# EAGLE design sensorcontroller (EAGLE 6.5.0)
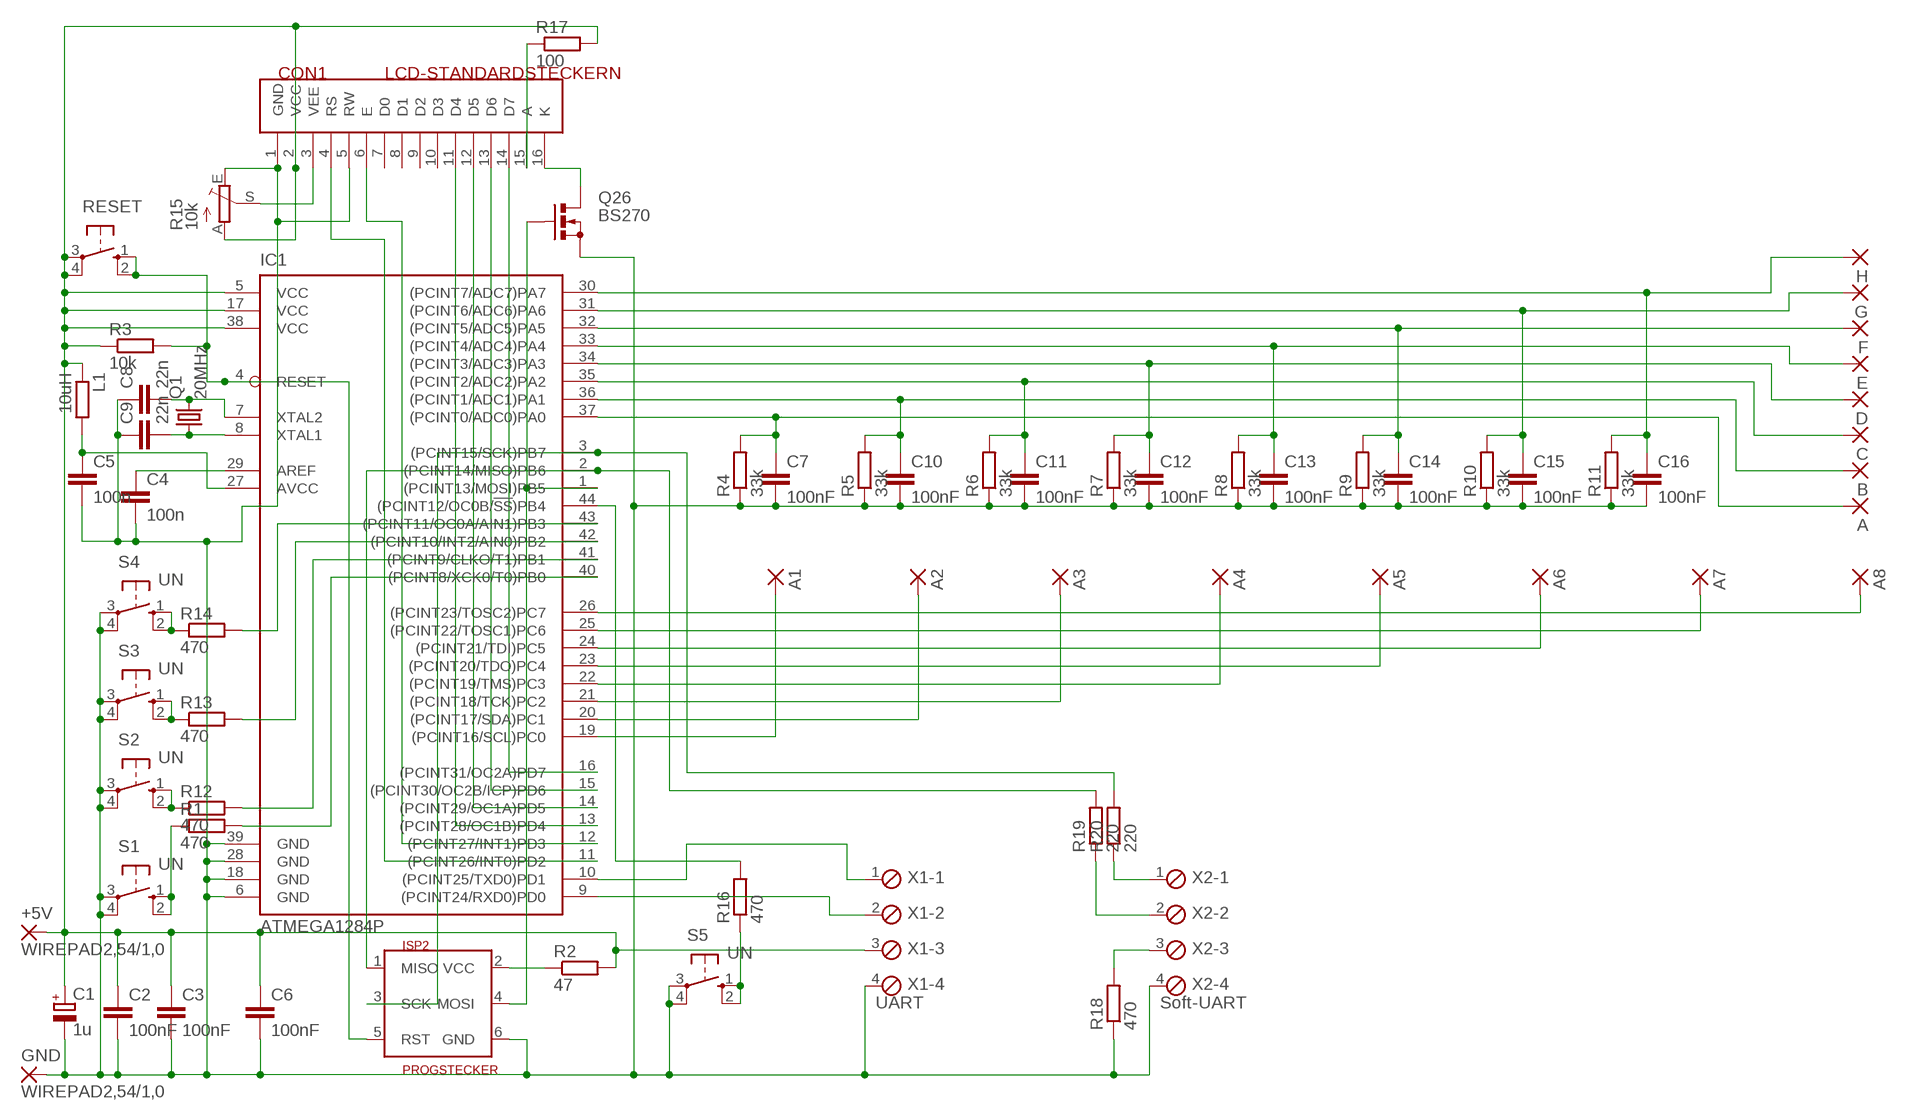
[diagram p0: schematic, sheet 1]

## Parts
+5V  WIREPAD2,54/1,0  [2,54/1,0]
A  WIREPAD2,15/1,0  [2,15/1,0]
A1  WIREPAD2,15/1,0  [2,15/1,0]
A2  WIREPAD2,15/1,0  [2,15/1,0]
A3  WIREPAD2,15/1,0  [2,15/1,0]
A4  WIREPAD2,15/1,0  [2,15/1,0]
A5  WIREPAD2,15/1,0  [2,15/1,0]
A6  WIREPAD2,15/1,0  [2,15/1,0]
A7  WIREPAD2,15/1,0  [2,15/1,0]
A8  WIREPAD2,15/1,0  [2,15/1,0]
B  WIREPAD2,15/1,0  [2,15/1,0]
C  WIREPAD2,15/1,0  [2,15/1,0]
C1  1u  CPOL-EUE5-6  [E5-6]
C2  100nF  C-EU025-025X050  [C025-025X050]
C3  100nF  C-EU025-025X050  [C025-025X050]
C4  100n  C-EUC1206  [C1206]
C5  100n  C-EUC1206  [C1206]
C6  100nF  C-EU025-025X050  [C025-025X050]
C7  100nF  C-EUC1206  [C1206]
C8  22n  C-EUC1206  [C1206]
C9  22n  C-EUC1206  [C1206]
C10  100nF  C-EUC1206  [C1206]
C11  100nF  C-EUC1206  [C1206]
C12  100nF  C-EUC1206  [C1206]
C13  100nF  C-EUC1206  [C1206]
C14  100nF  C-EUC1206  [C1206]
C15  100nF  C-EUC1206  [C1206]
C16  100nF  C-EUC1206  [C1206]
CON1  LCD-STANDARDSTECKERN  [STECKER16]
D  WIREPAD2,15/1,0  [2,15/1,0]
E  WIREPAD2,15/1,0  [2,15/1,0]
F  WIREPAD2,15/1,0  [2,15/1,0]
G  WIREPAD2,15/1,0  [2,15/1,0]
GND  WIREPAD2,54/1,0  [2,54/1,0]
H  WIREPAD2,15/1,0  [2,15/1,0]
IC1  ATMEGA1284P  ATMEGA644A  [TQFP44]
ISP2  PROGSTECKER  ISP6N  [ISP6]
L1  10uH  R-EU_0204/7  [0204/7]
Q1  20MHz  CRYSTALHC49S  [HC49/S]
Q26  BS270  BS170  [SOT54E]
R1  470  R-EU_M1406  [M1406]
R2  47  R-EU_M1406  [M1406]
R3  10k  R-EU_M1406  [M1406]
R4  33k  R-EU_M1406  [M1406]
R5  33k  R-EU_M1406  [M1406]
R6  33k  R-EU_M1406  [M1406]
R7  33k  R-EU_M1406  [M1406]
R8  33k  R-EU_M1406  [M1406]
R9  33k  R-EU_M1406  [M1406]
R10  33k  R-EU_M1406  [M1406]
R11  33k  R-EU_M1406  [M1406]
R12  470  R-EU_M1406  [M1406]
R13  470  R-EU_M1406  [M1406]
R14  470  R-EU_M1406  [M1406]
R15  10k  TRIM_EU-CA6V  [CA6V]
R16  470  R-EU_M1406  [M1406]
R17  100  R-EU_0204/7  [0204/7]
R18  470  R-EU_M1406  [M1406]
R19  220  R-EU_M1406  [M1406]
R20  220  R-EU_M1406  [M1406]
RESET  10-XX  [B3F-10XX]
S1  UN  10-XX  [B3F-10XX]
S2  UN  10-XX  [B3F-10XX]
S3  UN  10-XX  [B3F-10XX]
S4  UN  10-XX  [B3F-10XX]
S5  UN  10-XX  [B3F-10XX]
X1  UART  MPT4  [4POL254]
X2  Soft-UART  MPT4  [4POL254]

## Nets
AVCC [dick]: C5.1 IC1.27(AVCC) L1.2
GND [dick]: C1.- C2.2 C3.2 C4.2 C5.2 C6.2 C7.2 C8.1 C9.1 C10.2 C11.2 C12.2 C13.2 C14.2 C15.2 C16.2 CON1.1(GND) CON1.5(RW) GND.1(P) IC1.6(GND) IC1.18(GND) IC1.28(GND) IC1.39(GND) ISP2.6(GND) Q26.S R4.1 R5.1 R6.1 R7.1 R8.1 R9.1 R10.1 R11.1 R15.E R18.1 S1.3(P) S1.4(P1) S2.3(P) S2.4(P1) S3.3(P) S3.4(P1) S4.3(P) S4.4(P1) S5.3(P) S5.4(P1) X1.4 X2.4
N$1: C8.2 IC1.7(XTAL2) Q1.2
N$2 [dick]: ISP2.2(VCC) R2.1
N$3: A.1(P) C7.1 IC1.37((PCINT0/ADC0)PA0) R4.2
N$4 [dick]: R1.1 S1.1(S) S1.2(S1)
N$5: C9.2 IC1.8(XTAL1) Q1.1
N$6: IC1.4(RESET) ISP2.5(RST) R3.2 RESET.1(S) RESET.2(S1)
N$7: C15.1 G.1(P) IC1.31((PCINT6/ADC6)PA6) R10.2
N$8: IC1.40((PCINT8/XCK0/T0)PB0) R1.2
N$9: B.1(P) C10.1 IC1.36((PCINT1/ADC1)PA1) R5.2
N$10 [dick]: C4.1 IC1.29(AREF)
N$11: A2.1(P) IC1.20((PCINT17/SDA)PC1)
N$12: IC1.1((PCINT13/MOSI)PB5) ISP2.4(MOSI) Q26.G
N$13 [dick]: R12.1 S2.1(S) S2.2(S1)
N$14: A3.1(P) IC1.21((PCINT18/TCK)PC2)
N$15: C14.1 F.1(P) IC1.32((PCINT5/ADC5)PA5) R9.2
N$16: C13.1 E.1(P) IC1.33((PCINT4/ADC4)PA4) R8.2
N$20: C12.1 D.1(P) IC1.34((PCINT3/ADC3)PA3) R7.2
N$21: A1.1(P) IC1.19((PCINT16/SCL)PC0)
N$25: C11.1 C.1(P) IC1.35((PCINT2/ADC2)PA2) R6.2
N$26: C16.1 H.1(P) IC1.30((PCINT7/ADC7)PA7) R11.2
N$27: A4.1(P) IC1.22((PCINT19/TMS)PC3)
N$31: A5.1(P) IC1.23((PCINT20/TDO)PC4)
N$35: A6.1(P) IC1.24((PCINT21/TDI)PC5)
N$39: A7.1(P) IC1.25((PCINT22/TOSC1)PC6)
N$43: A8.1(P) IC1.26((PCINT23/TOSC2)PC7)
N$52 [dick]: R13.1 S3.1(S) S3.2(S1)
N$53 [dick]: R14.1 S4.1(S) S4.2(S1)
N$54: IC1.41((PCINT9/CLKO/T1)PB1) R12.2
N$55: IC1.42((PCINT10/INT2/AIN0)PB2) R13.2
N$56: IC1.43((PCINT11/OC0A/AIN1)PB3) R14.2
N$57: CON1.3(VEE) R15.S
N$58: CON1.4(RS) IC1.11((PCINT26/INT0)PD2)
N$59: CON1.6(E) IC1.12((PCINT27/INT1)PD3)
N$60: CON1.11(D4) IC1.13((PCINT28/OC1B)PD4)
N$61: CON1.12(D5) IC1.14((PCINT29/OC1A)PD5)
N$62: CON1.13(D6) IC1.15((PCINT30/OC2B/ICP)PD6)
N$63: CON1.14(D7) IC1.16((PCINT31/OC2A)PD7)
N$64 [sehrdick]: CON1.16(K) Q26.D
N$65 [dick]: R16.1 S5.1(S) S5.2(S1)
N$66: IC1.44((PCINT12/OC0B/!SS!)PB4) R16.2
N$67 [sehrdick]: CON1.15(A) R17.1
N$68: IC1.9((PCINT24/RXD0)PD0) X1.2
N$69: IC1.10((PCINT25/TXD0)PD1) X1.1
N$70: R18.2 X2.3
N$71: R19.1 X2.2
N$72: R20.1 X2.1
RXD2: IC1.2((PCINT14/MISO)PB6) ISP2.1(MISO) R19.2
TXD2: IC1.3((PCINT15/SCK)PB7) ISP2.3(SCK) R20.2
VCC [dick]: +5V.1(P) C1.+ C2.1 C3.1 C6.1 CON1.2(VCC) IC1.5(VCC) IC1.17(VCC) IC1.38(VCC) L1.1 R2.2 R3.1 R15.A R17.2 RESET.3(P) RESET.4(P1) X1.3
Unconnected: CON1.7(D0) CON1.8(D1) CON1.9(D2) CON1.10(D3)

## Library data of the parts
+5V A A1-A8 B C D E F G GND H = wirepad:WIREPAD: Wire PAD connect wire on PCB
C1 = resistor:CPOL-EU: POLARIZED CAPACITOR, European symbol
C2-C16 = rcl:C-EU: CAPACITOR, European symbol
CON1 = 6_stecker:LCD-STANDARDSTECKER: Standard-Stecker fuer die meisten LCD-Module
IC1 = atmel:ATMEGA644: 8-bit Microcontroller with 64K Bytes In-System Programmable Flash Source: http://www.atmel.com/dyn/resources/prod_documents/doc2593.pdf; MPN: ATMEGA644PV-10AU; OC_FARNELL: 1455123; OC_NEWARK: 58M3748
ISP2 = stecker:ISP6: ISP-Stecker 6polig
L1 R1-R14 R16-R20 = rcl:R-EU_: RESISTOR, European symbol
Q1 = crystal:CRYSTAL: CRYSTAL
Q26 = transistor-small-signal:BS170: N-CHANNEL MOS FET
R15 = pot:TRIM_EU-: POTENTIOMETER
RESET S1-S5 = switch-omron:10-XX: OMRON SWITCH; MPN: B3F-1000; OC_FARNELL: 176432; OC_NEWARK: 36M3542
X1 X2 = con-phoenix-254:MPT4: PHOENIX CONNECTOR; OC_FARNELL: unknown; OC_NEWARK: unknown

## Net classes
1 dick: width 0.508 mm
2 sehrdick: width 1.016 mm

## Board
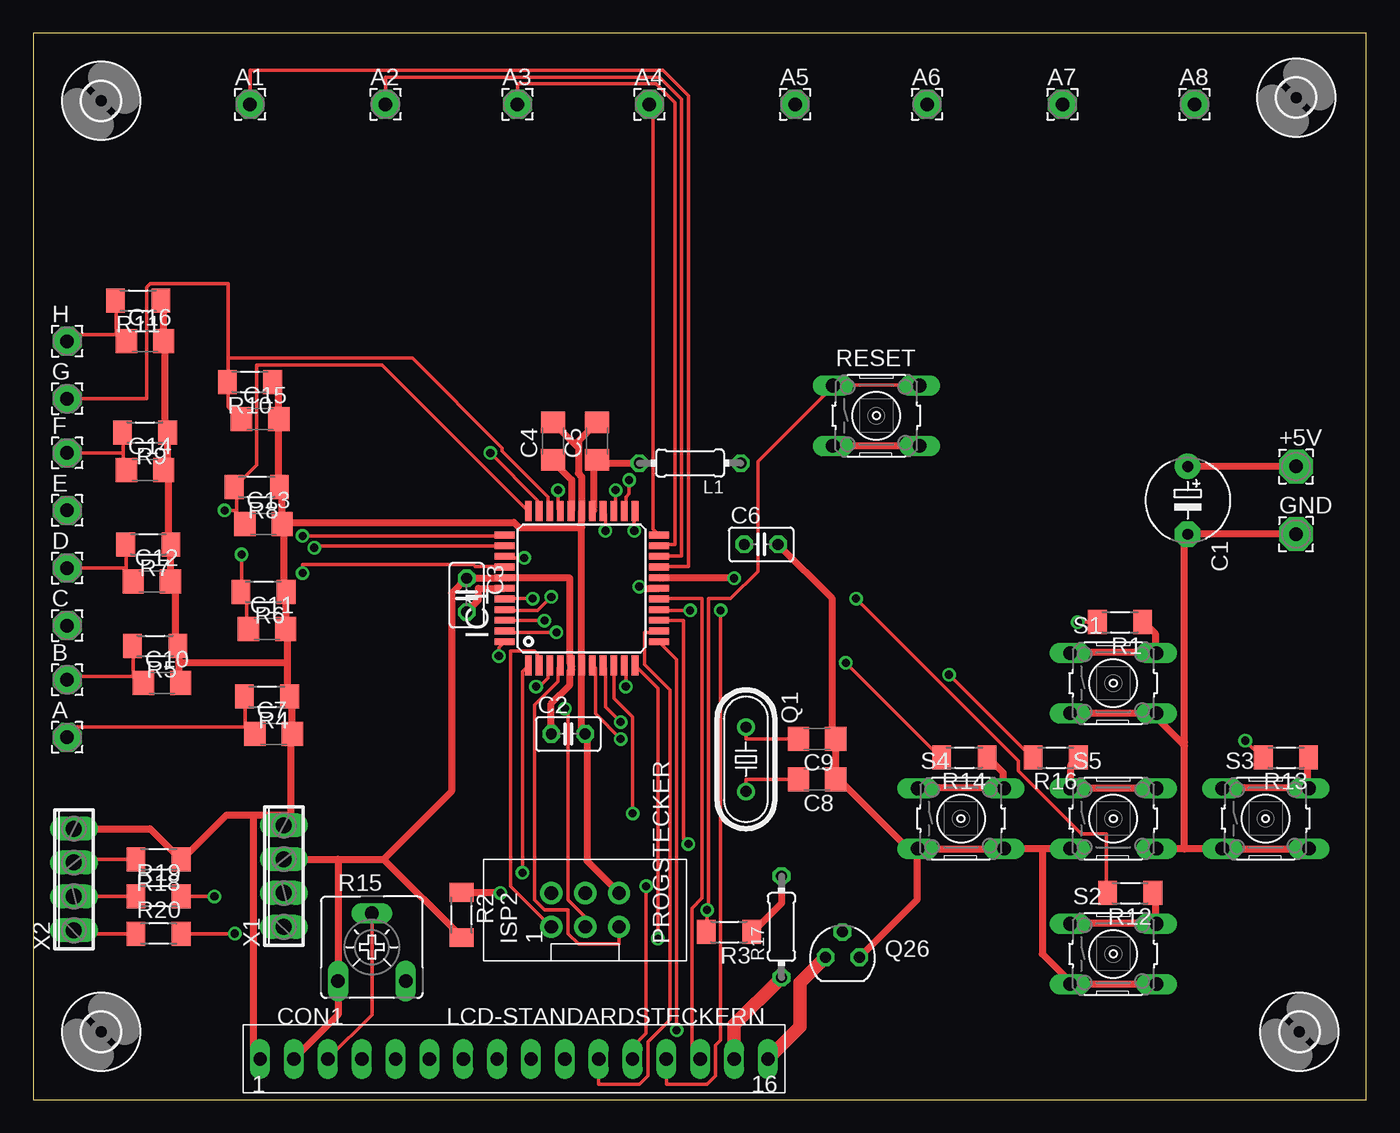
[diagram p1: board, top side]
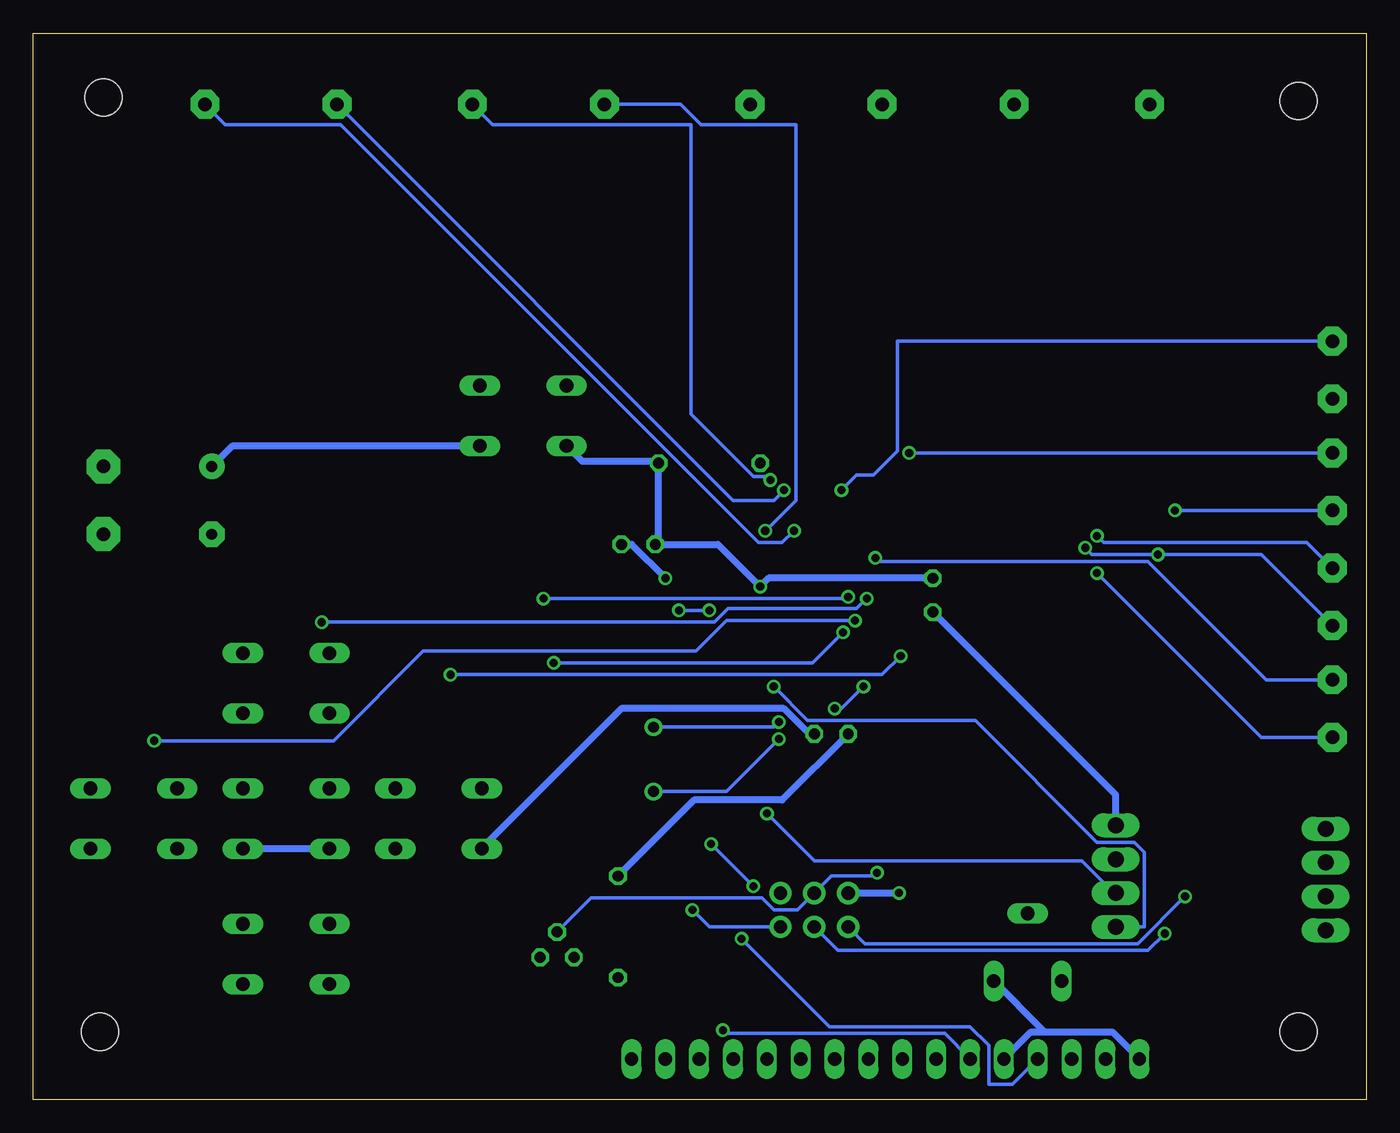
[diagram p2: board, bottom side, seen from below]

Size 100 x 80 mm. Coordinates in mm from the lower left corner, seen from the top.
Outline: 0,0 100,0 100,80 0,80 0,0
Copper layers (1*16): Top 0.035mm / dielectric 1.5mm / Bottom 0.035mm
Design rules "default": minimum track width 10mil, minimum drill 24mil, track to track 8mil, track to pad 8mil, pad to pad 8mil, via to via 8mil, smd to smd 8mil, copper to edge 40mil, drill to drill 8mil, minimum pad ring 10mil, minimum via ring 8mil, stop-mask expansion 4mil, vias tented up to drill 0mil, thermal gap 10mil

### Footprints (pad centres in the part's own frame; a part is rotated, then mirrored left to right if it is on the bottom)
2,54/1,0 = drill 1.016 pad 2.54 octagon: 1 0,0
2,15/1,0 = drill 1.016 pad 2.159 octagon: 1 0,0
E5-6 = drill 0.813 pad 1.905: + -2.54,0 | drill 0.813 pad 1.905 octagon: - 2.54,0
C025-025X050 = drill 0.813 octagon: 1 -1.27,0; 2 1.27,0
C1206 = smd 1.6 x 1.8: 1 -1.4,0; 2 1.4,0
STECKER16 = drill 1 long: 1 -17.78,0; 2 -15.24,0; 3 -12.7,0; 4 -10.16,0; 5 -7.62,0; 6 -5.08,0; 7 -2.54,0; 8 0,0; 9 2.54,0; 10 5.08,0; 11 7.62,0; 12 10.16,0; 13 12.7,0; 14 15.24,0; 15 17.78,0; 16 20.32,0
TQFP44 = smd 1.5 x 0.5: 1 -5.8,4; 2 -5.8,3.2; 3 -5.8,2.4; 4 -5.8,1.6; 5 -5.8,0.8; 6 -5.8,0; 7 -5.8,-0.8; 8 -5.8,-1.6; 9 -5.8,-2.4; 10 -5.8,-3.2; 11 -5.8,-4; 23 5.8,-4; 24 5.8,-3.2; 25 5.8,-2.4; 26 5.8,-1.6; 27 5.8,-0.8; 28 5.8,0; 29 5.8,0.8; 30 5.8,1.6; 31 5.8,2.4; 32 5.8,3.2; 33 5.8,4 | smd 0.5 x 1.5: 12 -4,-5.8; 13 -3.2,-5.8; 14 -2.4,-5.8; 15 -1.6,-5.8; 16 -0.8,-5.8; 17 0,-5.8; 18 0.8,-5.8; 19 1.6,-5.8; 20 2.4,-5.8; 21 3.2,-5.8; 22 4,-5.8; 34 4,5.8; 35 3.2,5.8; 36 2.4,5.8; 37 1.6,5.8; 38 0.8,5.8; 39 0,5.8; 40 -0.8,5.8; 41 -1.6,5.8; 42 -2.4,5.8; 43 -3.2,5.8; 44 -4,5.8
ISP6 = drill 1 pad 1.676: 1 -1.27,2.54; 2 1.27,2.54; 3 -1.27,0; 4 1.27,0; 5 -1.27,-2.54; 6 1.27,-2.54
0204/7 = drill 0.813 octagon: 1 -3.81,0; 2 3.81,0
HC49/S = drill 0.813: 1 -2.413,0; 2 2.413,0
SOT54E = drill 0.813 octagon: D -1.27,0; G 0,1.905; S 1.27,0
M1406 = smd 1.4 x 1.8: 1 -1.7,0; 2 1.7,0
CA6V = drill 1.016 long: A -2.54,-2.54; E 2.54,-2.54; S 0,2.54
B3F-10XX = drill 1.016 long: 1 -3.251,2.261; 2 3.251,2.261; 3 -3.251,-2.261; 4 3.251,-2.261
2,8 = hole 2.8: 0,0
4POL254 = drill 1.2 long: 1 -3.81,0; 2 -1.27,0; 3 1.27,0; 4 3.81,0

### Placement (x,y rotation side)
+5V  94.74,47.5 0 top
A  2.54,27.18 0 top
A1  16.26,74.68 0 top
A2  26.42,74.68 0 top
A3  36.32,74.68 0 top
A4  46.23,74.68 0 top
A5  57.15,74.68 0 top
A6  67.06,74.68 0 top
A7  77.22,74.68 0 top
A8  87.12,74.68 0 top
B  2.54,31.5 0 top
C  2.54,35.56 0 top
C1  86.61,44.96 270 top
C2  40.13,27.43 0 top
C3  32.51,37.85 270 top
C4  38.99,49.4 90 top
C5  42.29,49.4 90 top
C6  54.61,41.66 0 top
C7  18.03,27.43 0 top
C8  58.8,24 180 top
C9  58.8,27.05 180 top
C10  9.65,31.24 0 top
C11  17.53,35.31 0 top
C12  8.89,38.86 0 top
C13  17.27,43.18 0 top
C14  8.38,47.24 0 top
C15  17.02,51.05 0 top
C16  8.38,56.9 0 top
CON1  34.8,3.05 0 top
D  2.54,39.88 0 top
E  2.54,44.2 0 top
F  2.54,48.51 0 top
G  2.54,52.58 0 top
GND  94.74,42.42 0 top
H  2.54,56.9 0 top
IC1  41.15,38.35 90 top
ISP2  41.4,14.22 90 top
L1  49.28,47.75 180 top
Q1  53.47,25.53 270 top
Q26  60.71,10.67 0 top
R1  81.53,35.81 180 top
R2  32.13,13.84 270 top
R3  52.2,12.57 180 top
R4  17.53,30.23 180 top
R5  9.14,34.04 180 top
R6  17.27,38.1 180 top
R7  8.64,41.66 180 top
R8  16.76,45.97 180 top
R9  8.38,50.04 180 top
R10  16.26,53.85 180 top
R11  7.87,59.94 180 top
R12  82.3,15.49 180 top
R13  93.98,25.65 180 top
R14  69.85,25.65 180 top
R15  25.4,11.43 0 top
R16  76.71,25.65 180 top
R17  56.13,12.95 90 top
R18  9.4,18.03 180 top
R19  9.4,15.24 0 top
R20  9.4,12.45 0 top
RESET  63.25,51.31 0 top
S1  81.03,31.24 0 top
S2  81.03,10.92 0 top
S3  92.46,21.08 0 top
S4  69.6,21.08 0 top
S5  81.03,21.08 0 top
U$1  [2,8]  95,5.08 0 top
U$2  [2,8]  5.08,5.08 0 top
U$3  [2,8]  5.08,74.93 0 top
U$4  [2,8]  94.74,75.18 0 top
X1  18.8,16.76 90 top
X2  3.05,16.51 90 top

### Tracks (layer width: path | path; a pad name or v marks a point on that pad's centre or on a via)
AVCC
  Top 0.508: 42.04,44.2 IC1.27 42.04,44.45 42.04,47.62 42.29,47.88 C5.1 42.42,47.75 L1.2
GND  (via drill 0.61)
  Top 0.508: GND.1 C1.- 86.36,42.16 86.36,26.8 86.23,26.67 | S1.3 77.85,28.96 84.2,28.96 S1.4 84.2,28.7 86.23,26.67 | 86.36,18.8 89.15,18.8 S3.3 89.41,18.8 95.63,18.8 S3.4 | 86.36,18.8 84.33,18.8 S5.4 | 86.23,26.67 86.36,26.54 86.36,18.8 | 46.99,39.12 IC1.18 47.24,39.12 v52.58,39.12 | S2.4 84.2,8.64 77.85,8.64 S2.3 77.72,8.89 75.69,10.92 75.69,18.8 | 75.69,18.8 77.72,18.8 S5.3 | 75.69,18.8 72.9,18.8 S4.4 72.64,18.8 66.55,18.8 S4.3 | Q26.S 66.29,14.99 66.29,18.8 S4.3 | S4.3 66.17,18.29 60.45,24 C8.1 C9.1 60.07,27.18 59.94,27.3 59.94,37.59 C6.2 | 41.15,44.2 IC1.28 | IC1.28 41.15,46.74 40.89,46.99 40.89,49.02 | 40.89,49.02 40.89,49.4 C5.2 | C4.2 40.77,49.02 40.89,49.02 | 41.15,32.51 IC1.6 | IC1.6 41.15,27.69 C2.2 41.53,27.3 41.53,17.91 ISP2.6 | IC1.6 41.15,42.93 | 41.15,42.93 IC1.28 | R11.1 9.65,59.94 9.78,59.82 C16.2 9.91,56.77 9.91,50.16 R9.1 10.03,50.04 10.03,47.37 9.91,47.24 C14.2 10.03,47.12 10.16,46.99 10.16,41.78 R7.1 10.29,41.66 C12.2 10.41,38.73 10.67,38.48 10.67,34.16 R5.1 10.92,34.04 10.92,32.77 | 10.92,32.77 10.92,31.37 C10.2 | X2.4 8.76,20.32 11.05,18.03 R18.1 11.3,18.16 14.48,21.34 16.51,21.34 | 35.43,38.35 IC1.39 33.4,38.35 33.4,37.47 C3.2 | R10.1 18.03,53.85 18.41,53.47 C15.2 18.41,50.93 18.41,46.1 R8.1 18.54,45.97 18.67,45.85 C13.2 | C13.2 18.8,43.05 18.8,38.23 R6.1 18.92,38.1 C11.2 19.05,35.18 19.05,32.77 | 19.05,32.77 19.05,30.35 R4.1 19.3,30.23 19.43,30.1 C7.2 19.3,27.3 19.3,21.08 X1.4 19.18,21.34 16.51,21.34 | CON1.1 16.51,3.56 16.51,21.34 | 19.05,32.77 10.92,32.77 | 41.15,42.93 36.45,42.93 36.07,43.31 18.8,43.31 C13.2
  Bottom 0.508: v52.58,39.12 55.12,41.66 C6.2 | S5.4 84.2,18.8 77.85,18.8 S5.3 | CON1.1 19.05,5.08 24.26,5.08 | 24.26,5.08 25.15,5.08 CON1.5 | R15.E 24.26,5.21 24.26,5.08 | C3.2 18.8,22.86 X1.4 | C2.2 41.78,27.43 43.69,29.34 55.88,29.34 66.29,18.92 S4.3
N$1  (via drill 0.61)
  Top 0.254: v44.07,27.05 42.16,28.96 42.16,32.38 42.04,32.51 IC1.7 | C8.2 53.47,24 Q1.2
  Bottom 0.254: v44.07,27.05 48.01,23.11 Q1.2
N$2  (via drill 0.61)
  Top 0.508: v35.05,15.49 32.13,15.49 R2.1
  Bottom 0.508: ISP2.2 v35.05,15.49
N$3  (via drill 0.61)
  Top 0.254: R4.2 15.88,30.23 15.88,28.07 16.51,27.43 C7.1 15.88,27.94 2.54,27.94 A.1 | v20.19,39.5 20.19,40.13 33.02,40.13 33.15,40.01 35.31,40.01 IC1.37
  Bottom 0.254: v20.19,39.5 7.87,27.18 A.1
N$4
  Top 0.508: R1.1 83.31,35.81 84.2,34.92 84.2,33.53 S1.2 83.95,33.53 77.85,33.53 S1.1
N$5  (via drill 0.61)
  Top 0.254: v44.07,28.32 42.93,29.46 42.93,32.38 42.8,32.51 IC1.8 | C9.2 53.47,27.05 Q1.1
  Bottom 0.254: v44.07,28.32 44.45,27.94 Q1.1
N$6  (via drill 0.61)
  Top 0.254: RESET.2 66.42,53.59 60.07,53.59 RESET.1 59.94,53.47 54.36,47.88 54.36,39.62 52.32,37.59 50.67,37.59 50.67,14.35 v50.55,14.22 50.55,12.57 R3.2 | ISP2.5 43.94,11.68 40.89,11.68 40.13,12.45 40.13,14.22 38.35,14.22 37.59,14.99 37.59,29.59 39.37,31.37 39.37,32.38 39.5,32.51 IC1.4
  Bottom 0.254: v50.55,14.22 49.28,12.95 ISP2.5
N$7
  Top 0.254: 14.61,55.63 28.45,55.63 35.18,48.9 35.18,48.64 38.61,45.21 38.61,44.32 38.73,44.2 IC1.31 | 14.61,53.85 14.61,55.63 | 14.61,53.85 14.61,51.94 15.49,51.05 C15.1 | 14.61,53.85 R10.2 | G.1 8.51,52.58 8.51,60.96 8.76,61.21 14.61,61.21 14.61,55.63
N$8  (via drill 0.61)
  Top 0.254: v37.47,37.59 35.43,37.59 IC1.40 | R1.2 v78.36,35.81
  Bottom 0.254: v37.47,37.59 38.23,36.83 47.88,36.83 48.9,35.81 v78.36,35.81
N$9  (via drill 0.61)
  Top 0.254: R5.2 7.49,34.04 7.49,31.88 8.13,31.24 C10.1 7.49,31.75 2.54,31.75 B.1 | v36.83,40.64 35.43,40.64 IC1.36
  Bottom 0.254: v36.83,40.64 36.58,40.39 16.38,40.39 7.49,31.5 B.1
N$10
  Top 0.508: IC1.29 40.39,44.2 40.39,46.48 38.99,47.88 C4.1
N$11
  Top 0.254: A2.1 26.42,76.71 46.99,76.71 48.64,75.06 48.64,40.77 46.99,40.77 IC1.20
N$12  (via drill 0.61)
  Top 0.254: v36.7,17.02 36.7,32.13 37.08,32.51 IC1.1
  Bottom 0.254: v36.7,17.02 36.96,16.76 40.13,16.76 ISP2.4 42.67,14.22 44.45,14.22 45.34,15.11 58.17,15.11 Q26.G
N$13
  Top 0.508: R12.1 84.07,15.49 84.2,15.37 84.2,13.21 S2.2 83.95,13.21 77.85,13.21 S2.1
N$14
  Top 0.254: A3.1 36.32,76.2 46.74,76.2 48.13,74.8 48.13,41.66 46.99,41.66 IC1.21
N$15  (via drill 0.61)
  Top 0.254: 6.73,48.51 6.73,50.04 R9.2 | 6.73,48.51 6.73,47.37 6.86,47.24 C14.1 | v34.29,48.51 37.85,44.96 37.85,44.2 IC1.32 | F.1 6.73,48.51
  Bottom 0.254: F.1 v34.29,48.51
N$16  (via drill 0.61)
  Top 0.254: IC1.33 37.08,44.2 26.16,55.12 16.76,55.12 16.76,47.62 15.11,45.97 R8.2 15.24,45.97 15.24,44.2 | 15.24,44.2 15.24,43.69 15.75,43.18 C13.1 | 15.24,44.2 v14.35,44.2
  Bottom 0.254: v14.35,44.2 E.1
N$20  (via drill 0.61)
  Top 0.254: 6.99,39.88 6.99,41.66 R7.2 | 6.99,39.88 6.99,39.24 7.37,38.86 C12.1 | v20.19,42.29 35.31,42.29 IC1.34 | D.1 6.99,39.88
  Bottom 0.254: v20.19,42.29 19.68,41.78 4.45,41.78 D.1
N$21
  Top 0.254: A1.1 16.26,77.22 47.24,77.22 49.15,75.31 49.15,40.01 46.99,40.01 IC1.19
N$25  (via drill 0.61)
  Top 0.254: 15.62,38.1 16,37.72 16,35.31 C11.1 | v21.08,41.4 21.08,41.53 35.31,41.53 IC1.35 | v15.62,40.89 15.62,38.1 | 15.62,38.1 R6.2
  Bottom 0.254: v21.08,41.4 20.57,40.89 v15.62,40.89 7.87,40.89 C.1
N$26  (via drill 0.61)
  Top 0.254: R11.2 6.22,59.94 6.22,57.53 6.86,56.9 C16.1 6.22,57.4 2.54,57.4 H.1 | v39.37,45.72 39.37,44.32 39.5,44.2 IC1.30
  Bottom 0.254: v39.37,45.72 38.23,46.86 36.96,46.86 35.18,48.64 35.18,56.9 H.1
N$27
  Top 0.254: A4.1 46.48,74.42 46.48,42.8 46.86,42.42 IC1.22
N$31  (via drill 0.61)
  Top 0.254: v45.09,42.67 45.09,44.07 IC1.23
  Bottom 0.254: v45.09,42.67 42.8,44.96 42.8,73.15 49.91,73.15 51.44,74.68 A5.1
N$35  (via drill 0.61)
  Top 0.254: v44.7,46.48 44.7,45.47 44.45,45.21 44.45,44.2 IC1.24
  Bottom 0.254: v44.7,46.48 44.96,46.74 45.97,46.74 50.67,51.44 50.67,73.15 65.53,73.15 A6.1
N$39  (via drill 0.61)
  Top 0.254: v43.69,45.72 43.69,44.32 43.56,44.2 IC1.25
  Bottom 0.254: v43.69,45.72 44.45,44.96 47.5,44.96 A7.1
N$43  (via drill 0.61)
  Top 0.254: v42.93,42.67 42.93,43.94 42.8,44.07 IC1.26
  Bottom 0.254: v42.93,42.67 43.81,41.78 45.59,41.78 76.96,73.15 85.6,73.15 A8.1
N$52
  Top 0.508: R13.1 95.63,25.65 95.63,23.37 S3.2 95.38,23.37 89.28,23.37 S3.1
N$53
  Top 0.508: R14.1 71.63,25.65 72.77,24.51 72.77,23.37 S4.2 72.52,23.37 66.42,23.37 S4.1
N$54  (via drill 0.61)
  Top 0.254: v38.86,37.72 37.85,36.7 35.43,36.7 IC1.41 | v61.72,37.59 73.91,25.4 73.91,24.64 78.61,19.94 80.52,19.94 80.52,15.49 R12.2
  Bottom 0.254: v38.86,37.72 38.99,37.59 v61.72,37.59
N$55  (via drill 0.61)
  Top 0.254: v38.35,35.94 35.43,35.94 IC1.42 | v90.93,26.92 92.2,25.65 R13.2
  Bottom 0.254: v38.35,35.94 48.01,35.94 50.29,33.66 70.74,33.66 77.47,26.92 v90.93,26.92
N$56  (via drill 0.61)
  Top 0.254: v39.24,35.05 35.43,35.05 IC1.43 | v60.96,32.77 68.07,25.65 R14.2
  Bottom 0.254: v39.24,35.05 41.53,32.77 v60.96,32.77
N$57
  Top 0.254: CON1.3 25.4,6.35 R15.S
N$58  (via drill 0.61)
  Top 0.254: v46.86,12.06 46.86,30.86 45.21,32.51 IC1.11
  Bottom 0.254: v46.86,12.06 40.26,5.46 29.72,5.46 28.32,4.06 28.32,1.14 26.54,1.14 CON1.4
N$59  (via drill 0.61)
  Top 0.254: v48.26,5.21 48.26,33.02 46.99,34.29 IC1.12
  Bottom 0.254: v48.26,5.21 48.01,4.95 31.62,4.95 CON1.6
N$60
  Top 0.254: CON1.11 42.42,1.14 45.47,1.14 46.1,1.78 46.1,4.32 47.75,5.97 47.75,30.73 45.85,32.64 45.85,35.05 46.86,35.05 IC1.13
N$61  (via drill 0.61)
  Top 0.254: v49.15,19.18 48.77,19.56 48.77,35.94 46.99,35.94 IC1.14 | v45.97,16 45.97,4.95 44.96,3.94 CON1.12
  Bottom 0.254: v45.97,16 v49.15,19.18
N$62  (via drill 0.61)
  Top 0.254: v49.28,36.7 46.99,36.7 IC1.15 | v51.56,36.7 51.56,4.45 51.18,4.06 51.18,1.78 50.55,1.14 47.5,1.14 CON1.13
  Bottom 0.254: v51.56,36.7 v49.28,36.7
N$63
  Top 0.254: CON1.14 49.4,3.68 49.4,14.35 50.16,15.11 50.16,37.59 46.99,37.59 IC1.16
N$64
  Top 1.016: Q26.D 57.53,8.76 57.53,5.46 CON1.16
N$65
  Top 0.508: R16.1 78.36,25.65 77.85,25.15 77.85,23.37 S5.1 78.11,23.37 84.2,23.37 S5.2
N$66  (via drill 0.61)
  Top 0.254: v34.92,33.27 34.92,33.91 35.31,34.29 IC1.44 | v68.71,31.88 74.93,25.65 R16.2
  Bottom 0.254: v34.92,33.27 36.32,31.88 v68.71,31.88
N$67
  Top 1.016: R17.1 52.58,5.59 CON1.15
N$68  (via drill 0.61)
  Top 0.254: v44.96,21.46 44.96,28.7 43.56,30.1 43.56,32.51 IC1.9
  Bottom 0.254: v44.96,21.46 41.4,17.91 21.34,17.91 18.92,15.49 X1.2
N$69  (via drill 0.61)
  Top 0.254: v44.45,30.99 44.45,32.51 IC1.10
  Bottom 0.254: v44.45,30.99 41.91,28.45 29.34,28.45 20.19,19.3 17.4,19.3 16.64,18.54 16.64,12.95 X1.1
N$70
  Top 0.254: R18.2 3.05,18.03 X2.3
N$71
  Top 0.254: X2.2 R19.1
N$72
  Top 0.254: R20.1 3.05,12.45 X2.1
RXD2  (via drill 0.61)
  Top 0.254: ISP2.1 35.81,16 35.81,33.66 37.59,33.66 37.85,33.4 37.85,32.64 IC1.2 | v13.59,15.24 R19.2
  Bottom 0.254: v13.59,15.24 17.14,11.68 37.59,11.68 ISP2.1
TXD2  (via drill 0.61)
  Top 0.254: v37.72,30.99 37.97,30.99 38.61,31.62 38.61,32.38 38.73,32.51 IC1.3 | v39.88,29.34 40.13,29.08 40.13,14.99 41.4,13.72 ISP2.3 | v15.11,12.45 R20.2
  Bottom 0.254: v37.72,30.99 39.37,29.34 v39.88,29.34 | v15.11,12.45 16.38,11.18 39.62,11.18 ISP2.3
VCC  (via drill 0.61)
  Top 0.508: +5V.1 C1.+ | RESET.3 60.07,49.02 66.42,49.02 RESET.4 | 46.99,38.35 IC1.17 45.47,38.35 v45.47,38.48 | CON1.2 22.86,6.35 R15.A 22.86,18.03 | 26.29,18.03 32.13,12.19 R2.2 | X1.3 22.86,18.03 | 22.86,18.03 26.29,18.03 | R17.2 56.13,14.73 53.98,12.57 R3.1 | 35.43,39.12 IC1.38 | IC1.38 35.18,39.12 C3.1 31.37,37.97 31.37,23.11 26.29,18.03 | 40.39,32.51 IC1.5 | C2.1 38.86,29.72 40.26,31.11 40.26,32.13 40.39,32.26 IC1.5 | IC1.38 35.69,39.12 40.26,39.12 40.26,32.77 IC1.5
  Bottom 0.508: RESET.3 59.94,49.02 58.8,47.88 53.21,47.88 L1.1 53.09,41.78 C6.1 48.64,41.66 v45.47,38.48 44.83,39.12 C3.1 | C1.+ 85.09,49.02 66.55,49.02 RESET.4 | R17.2 50.42,22.48 43.81,22.48 C2.1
